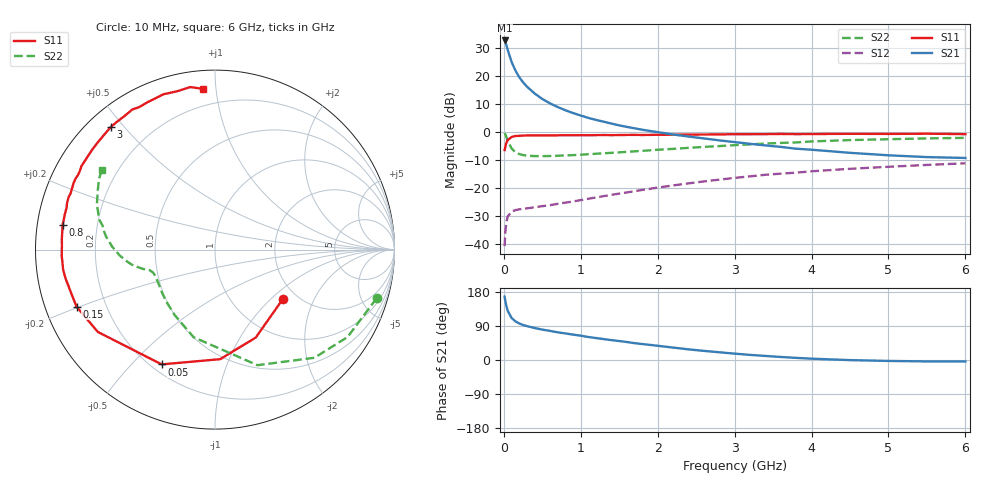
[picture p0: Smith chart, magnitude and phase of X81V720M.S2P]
! SIEMENS Small Signal Semiconductors
! BFP136W
! Si NPN RF Bipolar Junction Transistor in SOT343
! VCE = 1.75 V  IC = 20 mA
! Common Emitter S-Parameters:  September  1994
# GHz  S  MA  R  50
!  f  S11  S21  S12  S22
! GHz  MAG  ANG  MAG  ANG  MAG  ANG  MAG  ANG
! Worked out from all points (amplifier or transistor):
!   40 points, 10 MHz to 6 GHz, reference 50 ohm
!   highest |S21| = 32.5 dB at 10 MHz (marker M1)
!   |S21| within 3 dB of that: start of sweep to 46.7 MHz
!   unconditionally stable (mu >= 1): 841.6 MHz to 2.824 GHz
!   at 200 MHz: K = 0.34, MSG = 23.6 dB, |S12| = -27.8 dB
!   at 1.5 GHz: K = 1.18, MAG = 9.6 dB, |S12| = -22.1 dB
!   at 6 GHz: K = 1.00, MSG = 1.0 dB, |S12| = -11.3 dB
!   S11 on the Smith chart (normalised r, x): 10 MHz: 1.68, -1.19; 50 MHz: 0.24, -0.61; 150 MHz: 0.09, -0.20; 800 MHz: 0.08, +0.08; 3 GHz: 0.07, +0.46; 6 GHz: 0.10, +0.92
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0.01  0.4678 -36.4  42.27 167.1  0.009 76.5  0.9402 -16.8
0.02  0.54 -65.1  39.21 155.1  0.0164 66.7  0.8847 -33.4
0.03  0.6111 -87.3  36.09 145.2  0.0226 57.6  0.8186 -47.4
0.05  0.7051 -114.9  28.84 130.0  0.0305 43.6  0.6862 -69.8
0.1  0.798 -144.9  17.61 111.1  0.0372 29.6  0.5025 -103.7
0.15  0.8344 -157.6  12.32 102.0  0.0396 25.1  0.4276 -121.9
0.2  0.8386 -164.3  9.342 96.4  0.0409 23.8  0.3965 -133.3
0.25  0.8483 -169.2  7.566 92.4  0.0418 23.4  0.3807 -140.7
0.3  0.8533 -172.4  6.345 89.5  0.0425 24.2  0.3711 -145.8
0.4  0.8548 -177.8  4.787 84.4  0.0446 26.7  0.3647 -152.3
0.5  0.8532 178.6  3.818 80.2  0.0466 29.2  0.3642 -156.3
0.6  0.8553 176.1  3.185 76.8  0.0485 31.7  0.3662 -158.6
0.7  0.8571 173.0  2.741 73.1  0.0513 34.8  0.3699 -160.1
0.8  0.8604 170.8  2.399 70.1  0.0538 37.1  0.3747 -161.1
1.1  0.8593 164.1  1.75 60.6  0.0632 43.0  0.394 -163.3
1.5  0.8661 157.1  1.289 50.0  0.0781 48.7  0.4255 -165.9
2.2  0.8784 144.4  0.886 32.8  0.1092 51.1  0.4908 -171.9
3  0.8969 130.3  0.649 16.8  0.149 47.8  0.5713 178.6
3.2  0.8977 127.0  0.604 13.5  0.1585 46.4  0.5899 175.9
4.5  0.9118 108.3  0.417 -0.3  0.2162 35.1  0.7043 159.1
5.5  0.9162 98.7  0.35 -3.7  0.2537 26.8  0.755 149.0
6  0.8981 94.3  0.338 -3.9  0.2712 22.2  0.7719 144.9
